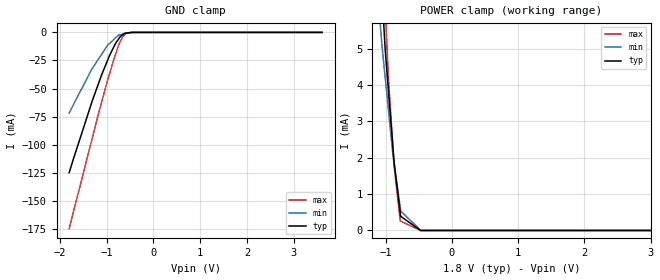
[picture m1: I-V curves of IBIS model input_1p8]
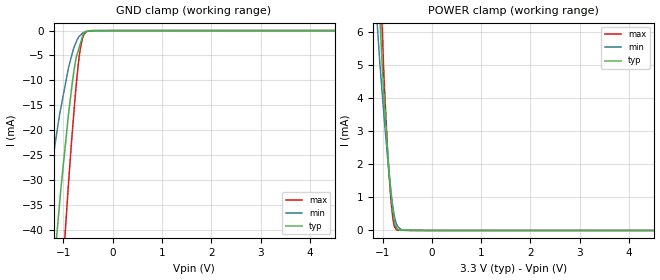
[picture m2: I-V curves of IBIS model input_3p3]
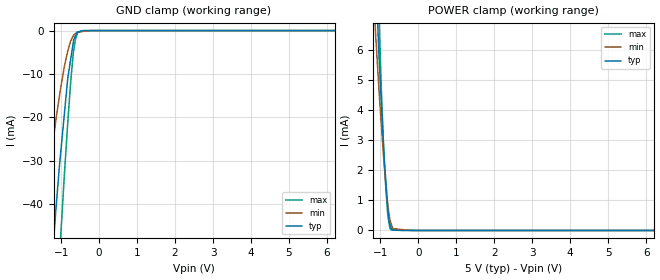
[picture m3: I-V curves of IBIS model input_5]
|Texas Instruments Incorporated
| Single Channel 16-Bit, Low Noise, Voltage Output Digital-to-Analog Converter
| Marketing part#   Digital Voltage Range   Package-type   #pins
| DAC8881SRGER   1.7V - 5.5V   VQFN   24
| DAC8881SRGERG4   1.7V - 5.5V   VQFN   24
| DAC8881SRGET   1.7V - 5.5V   VQFN   24
| DAC8881SRGETG4   1.7V - 5.5V   VQFN   24
[IBIS Ver]   3.2
[File name]   dac8881.ibs
|SIMDE Ver   V3.0 - 201101 - RHL4 - Build 457
[File Rev]   1.0
[Date]   9/14/2011
[Source]
| Texas Instruments Incorporated.
| Analog-eLab Design Center, HPA
| 12500 TI Blvd
| Dallas, TX -75243
| e-mail: elab_scm_ibis@list.ti.com
[Notes]   Revision History:
| Rev 1.0: 9/14/2011
| - Initial version of the model
| - Model generated from simulations in TISPICE
| - Model matched to SPICE simulation
| - C_comp although listed in numerical order of value are
|   obtained from varying PVT conditions. For PVT conditions for
|   each specific value refer the buffer description under
|   respective [Model]. IBIS model user is responsible for using
|   appropriate C_comp to simulate for Signal Integrity.
| - Model names with a trailing _1p8 contains the model for
|   1.8V [1.71V and 1.89V].Model names with a trailing _3p3
|   contains the model for 3.3V [3.0V and 3.6V]. Model names with
|   a trailing _5 contains the model for 5.0V [4.5V and 5.5V].
[Disclaimer]
| This model is designed as an aid for customers of Texas Instruments.
| TI and its licensors and suppliers make no warranties, either expressed
| or implied, with respect to this  model, including the warranties of
| merchantability or fitness for a particular purpose. The model is
| provided solely on an "as is" basis. The entire risk as to its quality
| and performance is with the customer.
[Copyright]
 (C) Copyright 2011 Texas Instruments Incorporated.All rights reserved.
|   DAC8881RGE
[Component]   DAC8881RGE
[Manufacturer]   TI
[Package]   |24 VQFN  -  RGE package
|   typ   min   max
R_pkg   0.04293   0.02082   0.04926
L_pkg   0.97310nH   0.59882nH   1.11595nH
C_pkg   0.33768pF   0.31938pF   0.36860pF
[Pin]  signal_name   model_name   R_pin   L_pin   C_pin
1   SCLK   INPUT   0.04857   1.09165nH  0.34123pF
2   SDI   INPUT   0.04590   1.02145nH  0.33121pF
3   _LDAC   INPUT   0.04501   0.99925nH  0.32966pF
4   AGND   GND   0.02275   0.68829nH  0.36903pF
5   AVDD   POWER   0.04599   1.02675nH  0.33245pF
6   VREFL-S   TERM   0.04926   1.11595nH  0.34350pF
7   VREFH-S   TERM   0.04482   0.99913nH  0.33499pF
8   VOUT   TERM   0.04012   0.87594nH  0.31938pF
9   RFB   TERM   0.04256   0.93975nH  0.32581pF
10   VREFL-F   TERM   0.02097   0.59882nH  0.36860pF
11   VREFH-F   TERM   0.02082   0.60800nH  0.36788pF
12   NC   NC   0.04948   1.12405nH  0.34889pF
13   NC   NC   0.05169   1.18185nH  0.34753pF
14   RSTSEL   INPUT   0.04895   1.10735nH  0.33699pF
15   GAIN   INPUT   0.04609   1.02965nH  0.33224pF
16   USB/_BTC   INPUT   0.04501   0.99931nH  0.32992pF
17   _RST   INPUT   0.04599   1.02375nH  0.33209pF
18   PDN   INPUT   0.04892   1.10085nH  0.34138pF
19   _CS   INPUT   0.04909   1.10345nH  0.34418pF
20   SDOSEL   INPUT   0.04414   0.97047nH  0.33220pF
21   DVDD   POWER   0.04321   0.94576nH  0.32581pF
22   DGND   GND   0.04325   0.94691nH  0.32459pF
23   SDO   SDO   0.04367   0.95798nH  0.32936pF
24   IOVDD   POWER   0.04771   1.06615nH  0.34118pF
25   THERMAL_PAD   NC   0.00008   0.00125nH  3.18442pF
|   Model Selectors
[Model Selector] INPUT
input_1p8   1.8V digital input
input_3p3   3.3V digital input
input_5   5.0V digital input
[Model Selector] SDO
sdo_1p8   1.8V digital 3-state
sdo_3p3   3.3V digital 3-state
sdo_5   5.0V digital 3-state
[Model Selector] TERM
term_1-8V  1.8V nominal termination
term_3-3V  3.3V nominal termination
term_5-0V  5.0V nominal termination
[Model] term_1-8V
Model_type Terminator
C_comp   1.0e-20F  1.0e-20F  1.0e-20F
|   typ   min   max
[Voltage Range]   1.8V   1.71V   1.89V
[POWER Clamp Reference]   1.8V   1.71V   1.89V
[GND Clamp Reference]   0V   0V   0V
|Ambient Temperature   25   105   -40
|Junction Temperature
[Temperature Range]   25   105   -40
[Model] term_3-3V
Model_type Terminator
C_comp   1.0e-20F  1.0e-20F  1.0e-20F
|   typ   min   max
[Voltage Range]   3.3V   3.0V   3.6V
[POWER Clamp Reference]   3.3V   3.0V   3.6V
[GND Clamp Reference]   0V   0V   0V
|Ambient Temperature   25   105   -40
|Junction Temperature
[Temperature Range]   25   105   -40
[Model] term_5-0V
Model_type Terminator
C_comp   1.0e-20F  1.0e-20F  1.0e-20F
|   typ   min   max
[Voltage Range]   5.0V   4.5V   5.5V
[POWER Clamp Reference]   5.0V   4.5V   5.5V
[GND Clamp Reference]   0V   0V   0V
|Ambient Temperature   25   105   -40
|Junction Temperature
[Temperature Range]   25   105   -40
| Models and submodels in the file (9): input_1p8 (Input), input_3p3 (Input), input_5 (Input), sdo_1p8 (3-state), sdo_3p3 (3-state), sdo_5 (3-state), term_1-8V (Terminator), term_3-3V (Terminator), term_5-0V (Terminator)
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|   input_1p8 Model
[Model]   input_1p8
Model_type   Input
Vinl = 0.3
Vinh = 1.5
|   typ   min   max
|   (nom PVT)   (fast PVT)   (slow PVT)
|C_comp from frequency sweep method (F=50MHz)
|Average
|C_comp   3.033e-12   2.462e-12   3.423e-12
|C_comp from LC tank measurement(L=1nH)
|Average
|Resonant Frequency(Hz)   3.330e+09   3.560e+09   3.160e+09
C_comp   2.287e-12   2.001e-12   2.539e-12
| Where nom  PVT is Nominal Process, 1.8V, 25C
|   Fast PVT is Strong Process,  1.89V, -40C
|   Slow PVT is Weak Process,   1.71V, 105C
[Voltage Range]   1.8   1.71   1.89
|Ambient Temperature   25   105   -40
|Junction Temperature
[Temperature Range]   25   105   -40
[Power Clamp Reference]   1.8   1.71   1.89
[GND Clamp Reference]   0   0   0
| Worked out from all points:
|   GND clamp passes 1 mA (typ) near -0.62 V on its own axis
|   POWER clamp passes 1 mA (typ) near -0.81 V on its own axis
[GND Clamp]
|   Voltage   I(typ)   I(min)   I(max)
-1.8V     -124.9mA   -71.68mA   -174.7mA
-1.32V    -62.68mA   -32.96mA   -96.26mA
-1.111V   -38.23mA   -19.73mA   -62.67mA
-981.5mV  -25.01mA   -11.57mA   -42.97mA
-943.2mV  -21.09mA   -10.06mA   -37.59mA
-811.8mV  -9.941mA   -4.963mA   -19.65mA
-733.3mV  -5.214mA   -2.238mA   -10.21mA
-703.8mV  -3.464mA   -1.993mA   -7.674mA
-657.7mV  -2.119mA   -1.61mA    -3.722mA
-584mV    -598.1uA   -997.6uA   -802.3uA
-391.6mV  -2.648uA   -7.888uA   -1.954uA
3.6V      0A         0A         0A
[POWER Clamp]
|   Voltage   I(typ)   I(min)   I(max)
-1.8V     36.74mA    28.17mA    45.65mA
-1.116V   8.437mA    6.435mA    10.91mA
-1.062V   6.714mA    5.209mA    8.352mA
-1.055V   6.486mA    5.056mA    8.065mA
-1.01V    5.037mA    4.233mA    6.236mA
-1.006V   4.938mA    4.168mA    6.09mA
-890.9mV  2.267mA    2.072mA    2.301mA
-869.4mV  1.81mA     1.792mA    1.71mA
-780.6mV  487.6uA    635uA      260.7uA
-774mV    389.8uA    549.4uA    255.2uA
-470.3mV  10.13nA    211.6nA    0A
3.6V      0A         0A         0A
|   input_3p3 Model
[Model]   input_3p3
Model_type   Input
Vinl = 0.6
Vinh = 2.1
|   typ   min   max
|   (nom PVT)   (fast PVT)   (slow PVT)
|C_comp from frequency sweep method (F=50MHz)
|Average
|C_comp   2.728e-12   2.201e-12   3.122e-12
|C_comp from LC tank measurement(L=1nH)
|Average
|Resonant Frequency(Hz)   3.470e+09   3.720e+09   3.270e+09
C_comp   2.106e-12   1.832e-12   2.371e-12
| Where nom  PVT is Nominal Process, 3.3V, 25C
|   Fast PVT is Strong Process,  3.6V, -40C
|   Slow PVT is Weak Process,   3V, 105C
[Voltage Range]   3.3   3   3.6
|Ambient Temperature   25   105   -40
|Junction Temperature
[Temperature Range]   25   105   -40
[Power Clamp Reference]   3.3   3   3.6
[GND Clamp Reference]   0   0   0
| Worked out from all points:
|   GND clamp passes 1 mA (typ) near -0.61 V on its own axis
|   POWER clamp passes 1 mA (typ) near -0.82 V on its own axis
[GND Clamp]
|   Voltage   I(typ)   I(min)   I(max)
-3.3V     -336.6mA   -225.3mA   -422.6mA
-1.429V   -76.08mA   -41.36mA   -113.5mA
-1.382V   -70.41mA   -37.84mA   -105.9mA
-1.224V   -51.13mA   -26.46mA   -80.38mA
-1.102V   -37.48mA   -18.48mA   -61.07mA
-1.049V   -31.67mA   -15.44mA   -53.35mA
-897.6mV  -16.92mA   -7.541mA   -30.9mA
-745.8mV  -5.602mA   -2.438mA   -11.63mA
-655.2mV  -2.611mA   -934.6uA   -3.566mA
-615.6mV  -1.304mA   -533.9uA   -1.664mA
-534.6mV  -127.5uA   -212.3uA   -222.7uA
6.6V      0A         0A         0A
[POWER Clamp]
|   Voltage   I(typ)   I(min)   I(max)
-3.3V     102.6mA    82.54mA    124.8mA
-1.155V   9.863mA    7.275mA    12.89mA
-1.096V   7.722mA    5.948mA    9.987mA
-1.044V   6.116mA    4.835mA    7.549mA
-1.003V   4.856mA    4.06mA     5.905mA
-972mV    4.121mA    3.468mA    4.647mA
-896.4mV  2.346mA    2.161mA    2.345mA
-838.8mV  1.276mA    1.299mA    1.085mA
-774mV    394.9uA    544.9uA    207.6uA
-712.8mV  62.54uA    176.6uA    15.22uA
-591mV    10.44uA    7.247uA    5.34uA
6.6V      0A         0A         0A
|   input_5 Model
[Model]   input_5
Model_type   Input
Vinl = 0.8
Vinh = 3.8
|   typ   min   max
|   (nom PVT)   (fast PVT)   (slow PVT)
|C_comp from frequency sweep method (F=50MHz)
|Average
|C_comp   2.503e-12   2.007e-12   2.891e-12
|C_comp from LC tank measurement(L=1nH)
|Average
|Resonant Frequency(Hz)   3.580e+09   3.850e+09   3.360e+09
C_comp   1.978e-12   1.711e-12   2.246e-12
| Where nom  PVT is Nominal Process, 5V, 25C
|   Fast PVT is Strong Process,  5.5V, -40C
|   Slow PVT is Weak Process,   4.5V, 105C
[Voltage Range]   5   4.5   5.5
|Ambient Temperature   25   105   -40
|Junction Temperature
[Temperature Range]   25   105   -40
[Power Clamp Reference]   5   4.5   5.5
[GND Clamp Reference]   0   0   0
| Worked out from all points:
|   GND clamp passes 1 mA (typ) near -0.61 V on its own axis
|   POWER clamp passes 1 mA (typ) near -0.82 V on its own axis
[GND Clamp]
|   Voltage   I(typ)   I(min)   I(max)
-5V       -580.3mA   -417.7mA   -700.9mA
-1.565V   -93.58mA   -52.23mA   -136mA
-1.375V   -69.33mA   -37.02mA   -104.7mA
-1.194V   -47.82mA   -24.27mA   -75.47mA
-1.017V   -28.63mA   -13.47mA   -48.28mA
-825mV    -10.93mA   -4.681mA   -21.13mA
-742.5mV  -6.258mA   -2.295mA   -11.19mA
-676.5mV  -2.521mA   -1.158mA   -5.015mA
-627mV    -1.306mA   -711.2uA   -2.11mA
-576mV    -368.7uA   -308.7uA   -764uA
-390.5mV  -7.899uA   -155.4uA   -1.819uA
10V       0A         0A         0A
[POWER Clamp]
|   Voltage   I(typ)   I(min)   I(max)
-5V       177.3mA    144.7mA    214.3mA
-1.14V    9.307mA    6.939mA    11.97mA
-1.127V   8.88mA     6.634mA    11.37mA
-1.045V   6.066mA    4.872mA    7.593mA
-1.026V   5.585mA    4.482mA    6.813mA
-924mV    3.004mA    2.638mA    3.087mA
-863.5mV  1.784mA    1.683mA    1.582mA
-803mV    731uA      863.7uA    507.9uA
-715mV    67.48uA    226.6uA    16.84uA
-670.5mV  13.62uA    63.4uA     15.79uA
-202.5mV  0A         0A         4.769uA
10V       0A         0A         0A
